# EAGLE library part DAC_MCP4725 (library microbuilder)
MCP4725 - 12-Bit I2C DAC with on-board EEPROM Settling Time: 6 µs 2.7-5.5V Supply 100kHz, 400kHz, 3.4 Mbps I²C EEPROM can be used to store a specific output voltage which will be set coming out of reset I²C Address: 1100 A2 A1 A0 A0 is set via the A0 pin, A2 and A1 are hard-wired on the chip depending on the model chosen: Part Number A2 A1 Code MCP4725A0T-E/CH 0 0 AJNN MCP4725A1T-E/CH 0 1 APNN MCP4725A2T-E/CH 1 0 AQNN MCP4725A3T-E/CH 1 1 ARNN
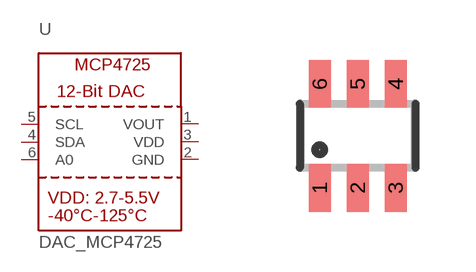
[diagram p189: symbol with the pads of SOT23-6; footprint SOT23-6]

Designator prefix U

## DAC_MCP4725  [SOT23-6]
1  VOUT  out
2  GND  pwr
3  VDD  pwr
4  SDA
5  SCL
6  A0  in

## Footprint SOT23-6 (pad centres in mm)
Small Outline Transistor - 6 Pin
smd 0.55 x 1.2: 1 -0.95,-1.3; 2 0,-1.3; 3 0.95,-1.3; 4 0.95,1.3; 5 0,1.3; 6 -0.95,1.3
